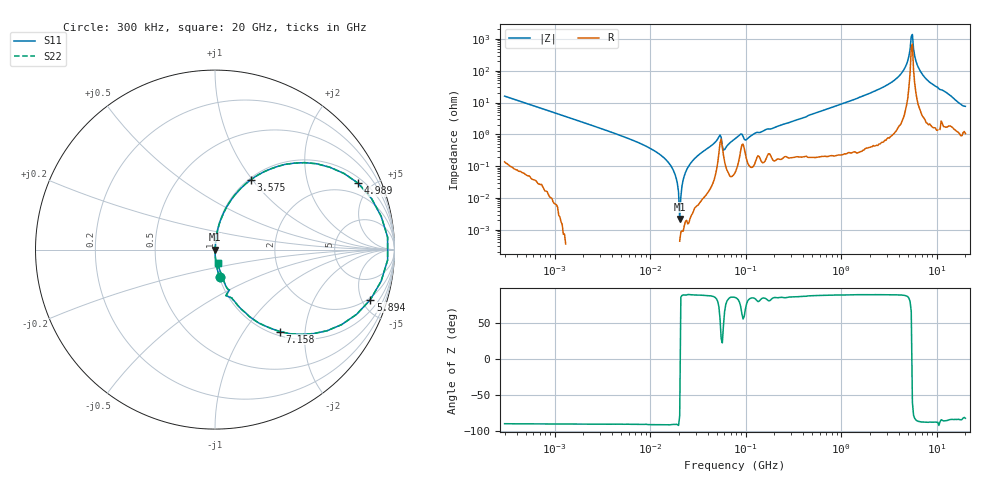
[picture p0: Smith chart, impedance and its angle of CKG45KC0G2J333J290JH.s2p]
! S-Parameter Data Generated by TDK Corporation
! Copyright(C) 2022 TDK Corporation.
! All Rights Reserved.
! TDK P/N: CKG45KC0G2J333J290JH (Multilayer Ceramic Chip Capacitor)
! Property: C=33nF
! Size(LxWxT): 5x3.5x2.9mm
! Model Type: s2p (Touchstone File Format Version 1.0)
! Frequency: DC=Yes Start=0.3MHz Stop=20000MHz 402points Log-sweep
! Model Generated on Apr. 15, 2022
! Port Assignments:
!  1 ---| |--- 2
! Applicable Conditions:
!  Temperature = 25 degC
!  DC Bias Voltage = 0 V
!  Small Signal Operation
! Terms and conditions regarding TDK Simulation Models
! (1)This simulation model is being provided solely for informational purposes. Please refer to the specifications of the products in terms of detailed characteristics of such products.
! (2)In no event shall TDK Corporation of any of its subsidiaries be liable for any loss or damage arising, directly or indirectly,
!  From any information contained in this simulation model, including, but not limited to loss or damages arising from any inaccuracies, omissions or errors in connection with such information.
! (3)Any and all copyrights on this simulation model are owned by TDK Corporation.
!  Duplication or redistribution of this simulation model without prior written permission from TDK Corporation is prohibited.
! (4)This simulation model is subject to any modification or change without any prior notice.
! (5)Neither TDK Corporation nor any of its subsidiaries shall make any warranty, express or implied,
!  Including but not limited to the correctness, implied warranties of merchantability and fitness for a particular purpose with respect to this simulation models.
! (6)The use of this simulation model shall be deemed to have consented to the terms and conditions hereof.
# Hz S MA R 50
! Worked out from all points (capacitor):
!   401 points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, 300 kHz to 20 GHz, reference 50 ohm
!   read as one part in series: C = 33.2 nF near 317.1 kHz
!   lowest |Z| = 2.19 mohm at 20.43 MHz (marker M1)
!   series resonance near 20.52 MHz, so ESL is about 1.8 nH
!   S11 on the Smith chart (normalised r, x): 300 kHz: 1.00, -0.32; 3.575 GHz: 1.02, +0.99; 4.989 GHz: 1.28, +4.18; 5.894 GHz: 1.80, -5.82; 7.158 GHz: 1.07, -1.48; 20 GHz: 1.02, -0.15
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300000  0.1575 -80.5  0.9862 9.1  0.9862 9.1  0.1575 -80.5
1928084  0.02456 -88.7  0.9997 1.4  0.9997 1.4  0.02456 -88.7
1.239169e7  0.002445 -90.7  1 0.1  1 0.1  0.002445 -90.7
1.681854e7  0.0009316 -90.8  1 0.1  1 0.1  0.0009316 -90.8
2.042709e7  2.193e-05 -78.5  1 0.0  1 0.0  2.193e-05 -78.5
2.413044e7  0.0007632 88.5  1 -0.0  1 -0.0  0.0007632 88.5
3.013307e7  0.001882 88.3  0.9999 -0.1  0.9999 -0.1  0.001882 88.3
5.250961e7  0.008308 71.9  0.9974 -0.5  0.9974 -0.5  0.008308 71.9
6.03306e7  0.003337 65.7  0.9986 -0.2  0.9986 -0.2  0.003337 65.7
7.964076e7  0.007712 84.0  0.9992 -0.4  0.9992 -0.4  0.007712 84.0
1.022524e8  0.006916 75.7  0.9983 -0.4  0.9983 -0.4  0.006916 75.7
4.978292e8  0.04319 85.0  0.9972 -2.5  0.9972 -2.5  0.04319 85.0
3.199522e9  0.3641 67.5  0.9243 -21.3  0.9243 -21.3  0.3641 67.5
3.575396e9  0.4385 62.8  0.8894 -26.0  0.8894 -26.0  0.4385 62.8
4.464803e9  0.6961 44.1  0.6964 -44.1  0.6964 -44.1  0.6961 44.1
4.98932e9  0.88 24.8  0.4206 -61.4  0.4206 -61.4  0.88 24.8
5.422764e9  0.9642 4.2  0.0798 -61.2  0.0798 -61.2  0.9642 4.2
5.893863e9  0.9095 -17.9  0.3097 64.3  0.3097 64.3  0.9095 -17.9
6.230452e9  0.8199 -30.7  0.5115 54.8  0.5115 54.8  0.8199 -30.7
7.158441e9  0.5825 -51.6  0.7849 35.6  0.7849 35.6  0.5825 -51.6
9.989315e9  0.2948 -70.4  0.943 17.1  0.943 17.1  0.2948 -70.4
2e10  0.07533 -77.7  0.9867 4.3  0.9867 4.3  0.07533 -77.7
